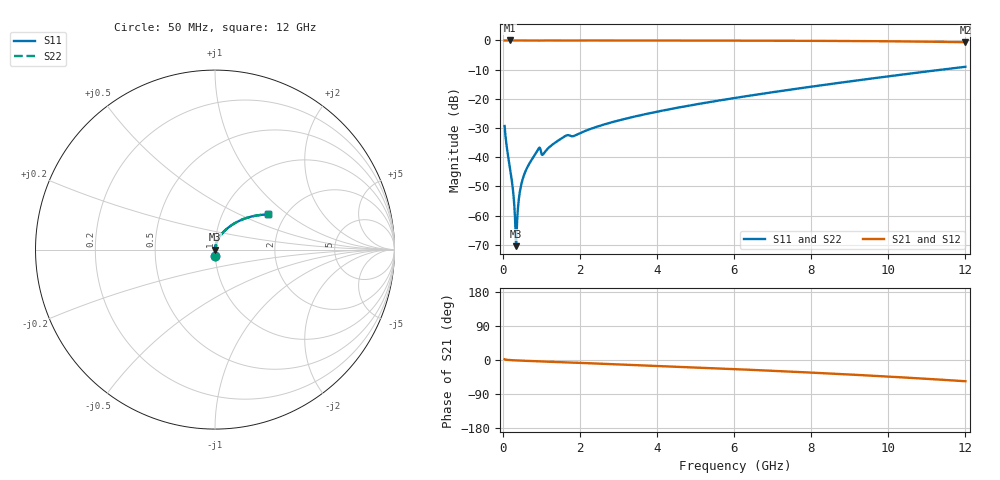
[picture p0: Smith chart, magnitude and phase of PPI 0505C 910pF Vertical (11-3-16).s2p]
# GHz S MA R 50
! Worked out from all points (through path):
!   1601 points, 50 MHz to 12 GHz, reference 50 ohm
!   highest |S21| = 0.00 dB at 184.4 MHz (marker M1); lowest = -0.6 dB at 12 GHz (marker M2)
!   group delay of S21, straight-line fit = 12.7 ps
!   lowest |S11| = -70.5 dB at 348.8 MHz (marker M3), VSWR 1.00, Z = 50 + j0.00188 ohm
!   |S11| at or under -10 dB: start of sweep to 11.39 GHz
!   |S22| runs from -70.5 to -9.0 dB; largest |S21 - S12| = 0
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0.05  0.03421 -87.9  0.9992 1.8  0.9992 1.8  0.03421 -87.9
0.1844375  0.006828 -88.1  0.9997 -0.2  0.9997 -0.2  0.006828 -88.1
0.2516563  0.003332 -86.0  0.9997 -0.6  0.9997 -0.6  0.003332 -86.0
0.3114062  0.001158 -76.5  0.9997 -0.9  0.9997 -0.9  0.001158 -76.5
0.34875  0.0002987 3.6  0.9997 -1.1  0.9997 -1.1  0.0002987 3.6
0.3860938  0.001101 72.5  0.9997 -1.2  0.9997 -1.2  0.001101 72.5
0.4533125  0.002742 81.6  0.9996 -1.5  0.9996 -1.5  0.002742 81.6
0.5354688  0.004565 83.7  0.9996 -1.9  0.9996 -1.9  0.004565 83.7
0.6624375  0.007183 84.4  0.9995 -2.4  0.9995 -2.4  0.007183 84.4
0.9014375  0.01293 80.5  0.9985 -3.5  0.9985 -3.5  0.01293 80.5
0.94625  0.01446 73.3  0.9966 -3.7  0.9966 -3.7  0.01446 73.3
1.058281  0.0114 76.5  0.998 -3.9  0.998 -3.9  0.0114 76.5
1.274875  0.01611 82.5  0.999 -4.8  0.999 -4.8  0.01611 82.5
1.610969  0.02279 79.2  0.9978 -6.2  0.9978 -6.2  0.02279 79.2
1.8425  0.02306 76.5  0.997 -6.9  0.997 -6.9  0.02306 76.5
2.044156  0.0265 79.7  0.9983 -7.7  0.9983 -7.7  0.0265 79.7
2.843313  0.03983 77.9  0.9982 -10.9  0.9982 -10.9  0.03983 77.9
4.038312  0.06077 73.5  0.9971 -15.7  0.9971 -15.7  0.06077 73.5
6.025  0.1035 65.3  0.9932 -24.1  0.9932 -24.1  0.1035 65.3
8.019156  0.162 56.2  0.985 -33.4  0.985 -33.4  0.162 56.2
10.01331  0.2432 45.8  0.9677 -43.8  0.9677 -43.8  0.2432 45.8
12  0.3538 33.6  0.9323 -56.1  0.9323 -56.1  0.3538 33.6
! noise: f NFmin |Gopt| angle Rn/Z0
0.05  0.0002963  0.8256  0.1886  0.0003571
1.372  0.003313  0.6205  4.062  0.001627
2.701  0.004847  0.5215  7.745  0.001767
4.031  0.006186  0.4638  11.15  0.001928
5.36  0.007671  0.4381  14.38  0.00223
6.682  0.009233  0.4267  17.42  0.002595
8.012  0.01094  0.4256  20.34  0.003045
9.341  0.01286  0.4334  23.16  0.003617
10.67  0.01507  0.4493  25.97  0.004368
12  0.0177  0.473  28.81  0.005387
